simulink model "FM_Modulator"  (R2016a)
settings: Solver=ode3  StartTime=0.0  StopTime=6  FixedStep=1/5000000  RelTol=1e-3

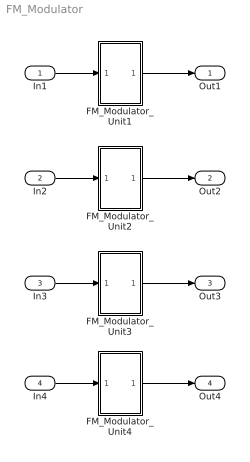
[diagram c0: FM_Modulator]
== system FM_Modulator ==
  In1 : Inport
  In2 : Inport  Port=2
  In3 : Inport  Port=3
  In4 : Inport  Port=4
  FM_Modulator_Unit1 : Subsystem
  FM_Modulator_Unit2 : Subsystem
  FM_Modulator_Unit3 : Subsystem
  FM_Modulator_Unit4 : Subsystem
  Out1 : Outport
  Out2 : Outport  Port=2
  Out3 : Outport  Port=3
  Out4 : Outport  Port=4
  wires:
  In1/1 -> FM_Modulator_Unit1/1(In1)
  FM_Modulator_Unit1/1(Out1) -> Out1/1
  In2/1 -> FM_Modulator_Unit2/1(In1)
  FM_Modulator_Unit2/1(Out1) -> Out2/1
  In3/1 -> FM_Modulator_Unit3/1(In1)
  FM_Modulator_Unit3/1(Out1) -> Out3/1
  In4/1 -> FM_Modulator_Unit4/1(In1)
  FM_Modulator_Unit4/1(Out1) -> Out4/1

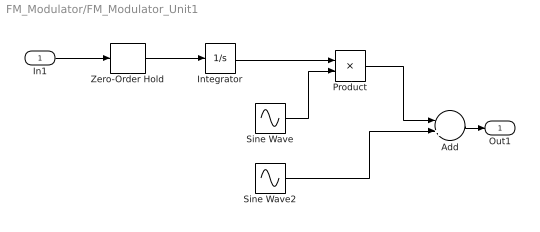
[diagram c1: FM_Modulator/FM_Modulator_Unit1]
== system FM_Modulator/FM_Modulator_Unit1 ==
  In1 : Inport
  Add : Sum  Inputs=-+
  Integrator : Integrator
  Product : Product
  Sine Wave : Sin  Frequency=500000*2*pi  Phase=-0.5*pi
  Sine Wave2 : Sin  Frequency=500000*2*pi
  Zero-Order Hold : ZeroOrderHold  SampleTime=1/5000000
  Out1 : Outport
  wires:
  Zero-Order Hold/1 -> Integrator/1
  In1/1 -> Zero-Order Hold/1
  Sine Wave/1 -> Product/2
  Sine Wave2/1 -> Add/2
  Product/1 -> Add/1
  Integrator/1 -> Product/1
  Add/1 -> Out1/1

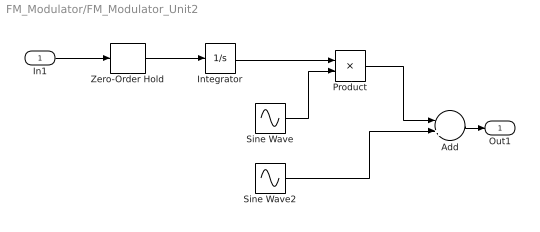
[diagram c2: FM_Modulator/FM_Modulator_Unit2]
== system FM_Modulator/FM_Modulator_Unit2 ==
  In1 : Inport
  Add : Sum  Inputs=-+
  Integrator : Integrator
  Product : Product
  Sine Wave : Sin  Frequency=500000*2*pi  Phase=-0.5*pi
  Sine Wave2 : Sin  Frequency=500000*2*pi
  Zero-Order Hold : ZeroOrderHold  SampleTime=1/5000000
  Out1 : Outport
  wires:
  Zero-Order Hold/1 -> Integrator/1
  In1/1 -> Zero-Order Hold/1
  Sine Wave/1 -> Product/2
  Sine Wave2/1 -> Add/2
  Product/1 -> Add/1
  Integrator/1 -> Product/1
  Add/1 -> Out1/1

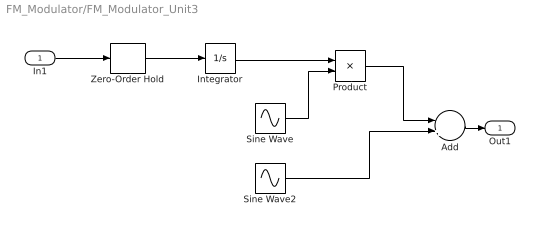
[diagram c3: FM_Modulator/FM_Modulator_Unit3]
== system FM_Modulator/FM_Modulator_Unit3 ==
  In1 : Inport
  Add : Sum  Inputs=-+
  Integrator : Integrator
  Product : Product
  Sine Wave : Sin  Frequency=500000*2*pi  Phase=-0.5*pi
  Sine Wave2 : Sin  Frequency=500000*2*pi
  Zero-Order Hold : ZeroOrderHold  SampleTime=1/5000000
  Out1 : Outport
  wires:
  Zero-Order Hold/1 -> Integrator/1
  In1/1 -> Zero-Order Hold/1
  Sine Wave/1 -> Product/2
  Sine Wave2/1 -> Add/2
  Product/1 -> Add/1
  Integrator/1 -> Product/1
  Add/1 -> Out1/1

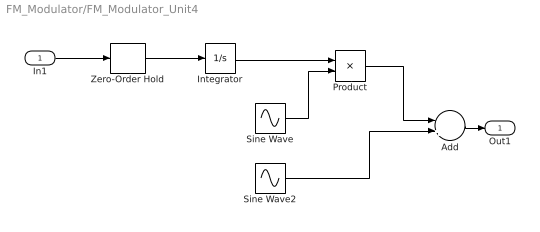
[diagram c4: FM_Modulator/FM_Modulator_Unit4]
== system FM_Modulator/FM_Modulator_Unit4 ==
  In1 : Inport
  Add : Sum  Inputs=-+
  Integrator : Integrator
  Product : Product
  Sine Wave : Sin  Frequency=500000*2*pi  Phase=-0.5*pi
  Sine Wave2 : Sin  Frequency=500000*2*pi
  Zero-Order Hold : ZeroOrderHold  SampleTime=1/5000000
  Out1 : Outport
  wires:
  Zero-Order Hold/1 -> Integrator/1
  In1/1 -> Zero-Order Hold/1
  Sine Wave/1 -> Product/2
  Sine Wave2/1 -> Add/2
  Product/1 -> Add/1
  Integrator/1 -> Product/1
  Add/1 -> Out1/1
